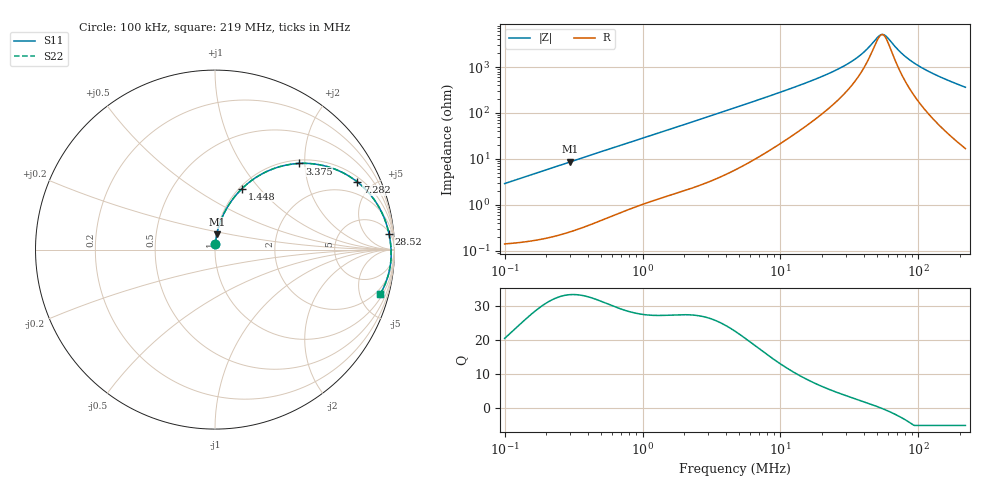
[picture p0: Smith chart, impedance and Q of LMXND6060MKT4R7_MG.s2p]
! LMXND6060MKT4R7_MG  S-PARAMETER MODEL  ( General Type )
! Model Generated by TAIYO YUDEN Corporation (http://www.ty-top.com)
! Version 1.0
! TAIYO YUDEN Control No. 191025NI43SB-FBB
! Copyright(c) 2019 TAIYO YUDEN CO.,LTD. All Rights Reserved.
! Product Description (link to TY-COMPAS)
! https://ds.yuden.co.jp/TYCOMPAS/or/detail?pn=LMXND6060MKT4R7MMG&u=M
! Products Name : Inductors
! Characteristics :
!  Inductance : 4.7 uH , SRF(min) : 36 MHz , DC Resistance(max) : 0.15 Ohm
!  Rated Current : Saturation :1600 mA , Temp Rise : 1550 mA
!  Case Size : 6.0 x 6.0 / 0.236 x 0.236 [mm/inch] , Thickness : 1.2 / 0.047 [mm/inch]
!  (Conditions: Temperature = 25 degC , DC Bias Current/Voltage = 0A / 0V)
! External Node Assignments :
!  1  o---GGG---o  2
! GND o---------o GND
! Frequency Range : 0.1MHz  -  218.972167MHz  [ 402 STEP ]
# MHz S RI R 50
! Freq[MHz].  S11 Real  S11 Imag  S21 Real  S21 Imag  S12 Real  S12 Imag  S22 Real  S22 Imag
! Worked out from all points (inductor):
!   401 points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, 100 kHz to 219 MHz, reference 50 ohm
!   read as one part in series: L = 4.62 uH near 103.9 kHz
!   highest Q = 33.5 at 299.2 kHz (marker M1), where L = 4.6 uH
!   self-resonance near 54.44 MHz
!   S11 on the Smith chart (normalised r, x): 100 kHz: 1.00, +0.06; 1.448 MHz: 1.03, +0.81; 3.375 MHz: 1.07, +1.88; 7.282 MHz: 1.24, +4.08; 28.52 MHz: 6, +20; 219 MHz: 1.34, -7.28
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0.1  0.00224 0.0289  0.9978 -0.0289  0.9978 -0.0289  0.00224 0.0289
0.29923  0.00995 0.0854  0.99 -0.0854  0.99 -0.0854  0.00995 0.0854
0.362673  0.0139 0.1029  0.9861 -0.1029  0.9861 -0.1029  0.0139 0.1029
0.76772  0.0523 0.2059  0.9477 -0.2059  0.9477 -0.2059  0.0523 0.2059
1.315317  0.1295 0.318  0.8705 -0.318  0.8705 -0.318  0.1295 0.318
1.448055  0.151 0.3402  0.849 -0.3402  0.849 -0.3402  0.151 0.3402
2.168481  0.2754 0.4289  0.7246 -0.4289  0.7246 -0.4289  0.2754 0.4289
3.374644  0.4699 0.4801  0.5301 -0.4801  0.5301 -0.4801  0.4699 0.4801
4.770297  0.633 0.4603  0.367 -0.4603  0.367 -0.4603  0.633 0.4603
7.282271  0.7935 0.3765  0.2065 -0.3765  0.2065 -0.3765  0.7935 0.3765
10.6976  0.885 0.281  0.115 -0.281  0.115 -0.281  0.885 0.281
16.97108  0.942 0.1781  0.058 -0.1781  0.058 -0.1781  0.942 0.1781
28.52239  0.9693 0.0886  0.0307 -0.0886  0.0307 -0.0886  0.9693 0.0886
33.91131  0.974 0.0636  0.026 -0.0636  0.026 -0.0636  0.974 0.0636
38.79729  0.9768 0.0451  0.0232 -0.0451  0.0232 -0.0451  0.9768 0.0451
52.77363  0.9807 0.00413  0.0193 -0.00413  0.0193 -0.00413  0.9807 0.00413
56.99291  0.9812 -0.00613  0.0188 0.00613  0.0188 0.00613  0.9812 -0.00613
61.54953  0.9814 -0.0165  0.0186 0.0165  0.0186 0.0165  0.9814 -0.0165
77.52404  0.9808 -0.049  0.0192 0.049  0.0192 0.049  0.9808 -0.049
99.54032  0.9768 -0.0878  0.0232 0.0878  0.0232 0.0878  0.9768 -0.0878
143.4391  0.9617 -0.1542  0.0383 0.1542  0.0383 0.1542  0.9617 -0.1542
218.9722  0.92 -0.2491  0.08 0.2491  0.08 0.2491  0.92 -0.2491
